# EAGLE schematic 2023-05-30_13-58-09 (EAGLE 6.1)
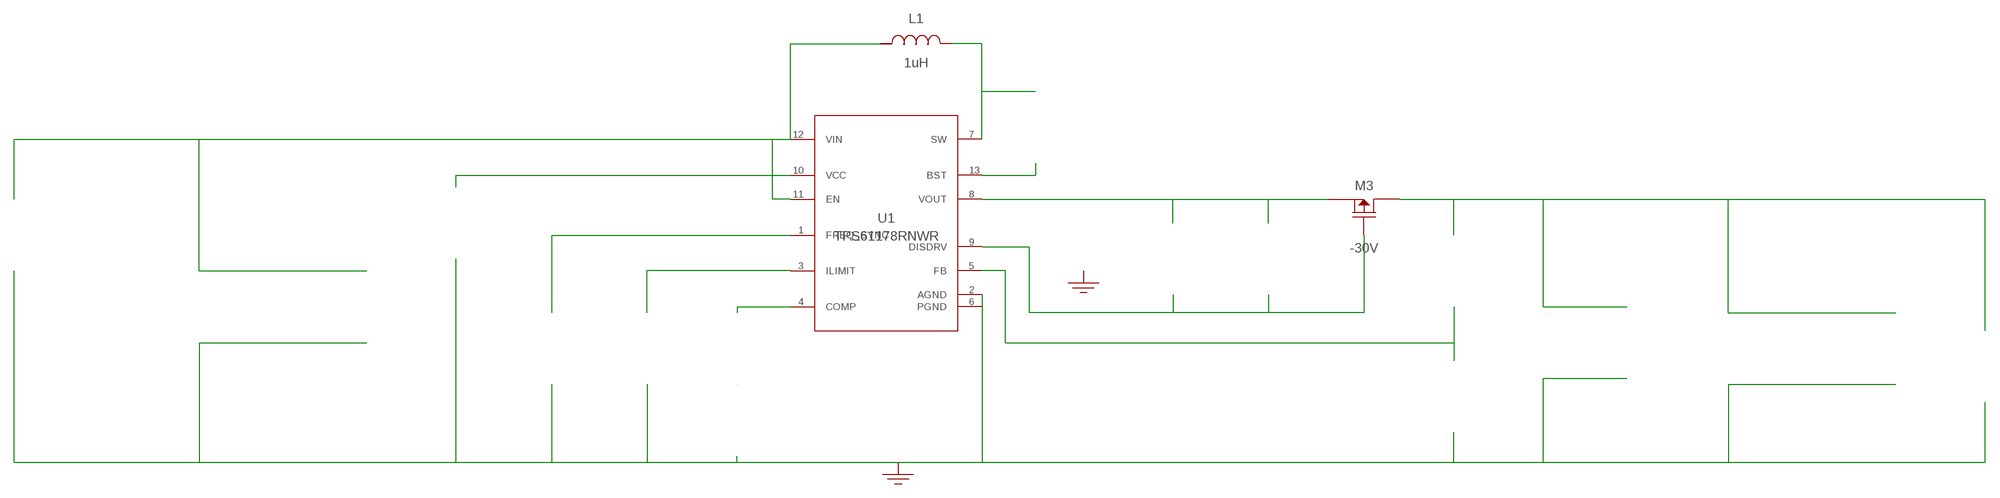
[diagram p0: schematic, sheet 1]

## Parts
CBOOT  100nF  08053C104KAT2A08053C104KAT2A  [0805]  (not placed on a sheet)
CCOMP  330pF  CL21C331JBANNNCCL21C331JBANNNC  [0805]  (not placed on a sheet)
CGATE  22nF  GRM155R71E223KA61DGRM155R71E223KA61D  [0402]  (not placed on a sheet)
CIN  22uF  GRM32ER61C226ME20LGRM32ER61C226ME20L  [1210]  (not placed on a sheet)
CIN_2  22uF  GRM32ER61C226ME20LGRM32ER61C226ME20L  [1210]  (not placed on a sheet)
CIN_3  22uF  GRM32ER61C226ME20LGRM32ER61C226ME20L  [1210]  (not placed on a sheet)
COUT  56uF  20SVPF56MX20SVPF56MX  [CAPSMT_62_E61]  (not placed on a sheet)
COUT1  10uF  CL32A106KBJNNNECL32A106KBJNNNE  [1210_270]  (not placed on a sheet)
COUT_2  56uF  20SVPF56MX20SVPF56MX  [CAPSMT_62_E61]  (not placed on a sheet)
COUT_3  56uF  20SVPF56MX20SVPF56MX  [CAPSMT_62_E61]  (not placed on a sheet)
COUTX  22uF  GRM32ER61E226KE15LGRM32ER61E226KE15L  [1210]  (not placed on a sheet)
COUTX_2  22uF  GRM32ER61E226KE15LGRM32ER61E226KE15L  [1210]  (not placed on a sheet)
CVCC  4.7uF  TMK212BJ475KG-TTMK212BJ475KG-T  [0805]  (not placed on a sheet)
GND  WB_GND  WB_GNDWB_GND  [WB_GND]
GND1  WB_GND  WB_GNDWB_GND  [WB_GND]
IOUT  WB_CURRENT_LOAD  WB_CURRENT_LOADWB_CURRENT_LOAD  [WB_CURRENT_LOAD]  (not placed on a sheet)
L1  1uH  IHLP3232DZER1R0M01IHLP3232DZER1R0M01  [IHLP-3232DZ]
M3  -30V  Si7135DPSi7135DP  [PowerPAK_SO-8]
RCOMP  86.6k  RC0201FR-0786K6LRC0201FR-0786K6L  [0201]  (not placed on a sheet)
RFBB  80.6k  CRCW040280K6FKEDCRCW040280K6FKED  [0402]  (not placed on a sheet)
RFBT  732k  CRCW0402732KFKEDCRCW0402732KFKED  [0402]  (not placed on a sheet)
RGATE  178k  CRCW0402178KFKEDCRCW0402178KFKED  [0402]  (not placed on a sheet)
RILIM  56.2k  RC0201FR-0756K2LRC0201FR-0756K2L  [0201]  (not placed on a sheet)
RT  412k  CRCW0402412KFKEDCRCW0402412KFKED  [0402]  (not placed on a sheet)
U1  TPS61178RNWR  TPS61178RNWRTPS61178RNWR  [RNW0013A]
VIN  WB_BATTERY  WB_BATTERYWB_BATTERY  [WB_BATTERY]  (not placed on a sheet)
Unconnected: CBOOT.1 CBOOT.2 CCOMP.1 CCOMP.2 CGATE.1 CGATE.2 CIN.1 CIN.2 CIN_2.1 CIN_2.2 CIN_3.1 CIN_3.2 COUT1.1 COUT1.2 COUT.1(+) COUT.2(-) COUT_2.1(+) COUT_2.2(-) COUT_3.1(+) COUT_3.2(-) COUTX.1 COUTX.2 COUTX_2.1 COUTX_2.2 CVCC.1 CVCC.2 GND1.1 GND.1 IOUT.1(+) IOUT.2(-) L1.1 L1.2 M3.1(Source) M3.2(Source) M3.3(Source) M3.4(Gate) M3.5(Drain) M3.6(Drain) M3.7(Drain) M3.8(Drain) M3.9(Drain) RCOMP.1 RCOMP.2 RFBB.1 RFBB.2 RFBT.1 RFBT.2 RGATE.1 RGATE.2 RILIM.1 RILIM.2 RT.1 RT.2 U1.1(FREQ_SYNC) U1.3(ILIMIT) U1.4(COMP) U1.5(FB) U1.9(DISDRV) U1.11(EN) VIN.1(+) VIN.2(-)

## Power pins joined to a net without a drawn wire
AGND: U1.2(AGND)
BST: U1.13(BST)
PGND: U1.6(PGND)
SW: U1.7(SW)
VCC: U1.10(VCC)
VIN: U1.12(VIN)
VOUT: U1.8(VOUT)

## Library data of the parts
CBOOT = AcceleratedDesigns_Lib:08053C104KAT2A; Manufacturer_Part_Number: 08053C104KAT2A; Vendor: AVX
CCOMP = AcceleratedDesigns_Lib:CL21C331JBANNNC; Manufacturer_Part_Number: CL21C331JBANNNC; Vendor: Samsung Electro-Mechanics
CGATE = AcceleratedDesigns_Lib:GRM155R71E223KA61D; Manufacturer_Part_Number: GRM155R71E223KA61D; Vendor: MuRata
CIN CIN_2 CIN_3 = AcceleratedDesigns_Lib:GRM32ER61C226ME20L; Manufacturer_Part_Number: GRM32ER61C226ME20L; Vendor: MuRata
COUT COUT_2 COUT_3 = AcceleratedDesigns_Lib:20SVPF56MX; Manufacturer_Part_Number: 20SVPF56MX; Vendor: Panasonic
COUT1 = AcceleratedDesigns_Lib:CL32A106KBJNNNE; Manufacturer_Part_Number: CL32A106KBJNNNE; Vendor: Samsung Electro-Mechanics
COUTX COUTX_2 = AcceleratedDesigns_Lib:GRM32ER61E226KE15L; Manufacturer_Part_Number: GRM32ER61E226KE15L; Vendor: MuRata
CVCC = AcceleratedDesigns_Lib:TMK212BJ475KG-T; Manufacturer_Part_Number: TMK212BJ475KG-T; Vendor: Taiyo Yuden
GND GND1 = AcceleratedDesigns_Lib:WB_GND; Manufacturer_Part_Number: WB_GND
IOUT = AcceleratedDesigns_Lib:WB_CURRENT_LOAD; Manufacturer_Part_Number: WB_CURRENT_LOAD
L1 = AcceleratedDesigns_Lib:IHLP3232DZER1R0M01; Manufacturer_Part_Number: IHLP3232DZER1R0M01; Vendor: Vishay-Dale
M3 = AcceleratedDesigns_Lib:Si7135DP; Manufacturer_Part_Number: Si7135DP; Vendor: Vishay-Siliconix
RCOMP = AcceleratedDesigns_Lib:RC0201FR-0786K6L; Manufacturer_Part_Number: RC0201FR-0786K6L; Vendor: Yageo America
RFBB = AcceleratedDesigns_Lib:CRCW040280K6FKED; Manufacturer_Part_Number: CRCW040280K6FKED; Vendor: Vishay-Dale
RFBT = AcceleratedDesigns_Lib:CRCW0402732KFKED; Manufacturer_Part_Number: CRCW0402732KFKED; Vendor: Vishay-Dale
RGATE = AcceleratedDesigns_Lib:CRCW0402178KFKED; Manufacturer_Part_Number: CRCW0402178KFKED; Vendor: Vishay-Dale
RILIM = AcceleratedDesigns_Lib:RC0201FR-0756K2L; Manufacturer_Part_Number: RC0201FR-0756K2L; Vendor: Yageo America
RT = AcceleratedDesigns_Lib:CRCW0402412KFKED; Manufacturer_Part_Number: CRCW0402412KFKED; Vendor: Vishay-Dale
U1 = AcceleratedDesigns_Lib:TPS61178RNWR; Manufacturer_Part_Number: TPS61178RNWR
VIN = AcceleratedDesigns_Lib:WB_BATTERY; Manufacturer_Part_Number: WB_BATTERY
